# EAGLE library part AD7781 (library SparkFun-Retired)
20-Bit, Pin-Programmable, Ultralow Power Sigma-Delta ADC Dead Prototype: IC-10476
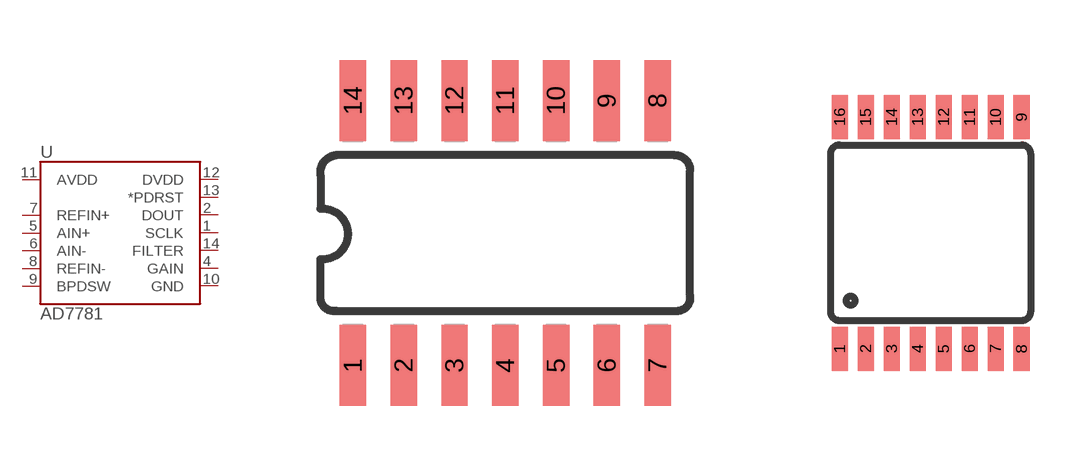
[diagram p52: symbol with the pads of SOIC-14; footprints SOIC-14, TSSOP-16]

Designator prefix U

## AD7781CRZ  [SOIC-14]
1  SCLK
2  DOUT
4  GAIN
5  AIN+
6  AIN-
7  REFIN+
8  REFIN-
9  BPDSW
10  GND
11  AVDD
12  DVDD
13  *PDRST
14  FILTER

## AD7781CRUZ  [TSSOP-16]
2  SCLK
3  DOUT
5  GAIN
6  AIN+
7  AIN-
8  REFIN+
9  REFIN-
10  BPDSW
11  GND
12  AVDD
13  DVDD
14  *PDRST
15  FILTER

## Footprint SOIC-14 (pad centres in mm)
smd 0.66 x 2.032: 1 -4.445,-3.315; 2 -3.175,-3.315; 3 -1.905,-3.315; 4 -0.635,-3.315; 5 0.635,-3.315; 6 1.905,-3.315; 7 3.175,-3.315; 8 3.175,3.315; 9 1.905,3.315; 10 0.635,3.315; 11 -0.635,3.315; 12 -1.905,3.315; 13 -3.175,3.315; 14 -4.445,3.315

## Footprint TSSOP-16 (pad centres in mm)
smd 0.4 x 1.1: 1 -2.275,-2.9; 2 -1.625,-2.9; 3 -0.975,-2.9; 4 -0.325,-2.9; 5 0.325,-2.9; 6 0.975,-2.9; 7 1.625,-2.9; 8 2.275,-2.9; 9 2.275,2.9; 10 1.625,2.9; 11 0.975,2.9; 12 0.325,2.9; 13 -0.325,2.9; 14 -0.975,2.9; 15 -1.625,2.9; 16 -2.275,2.9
